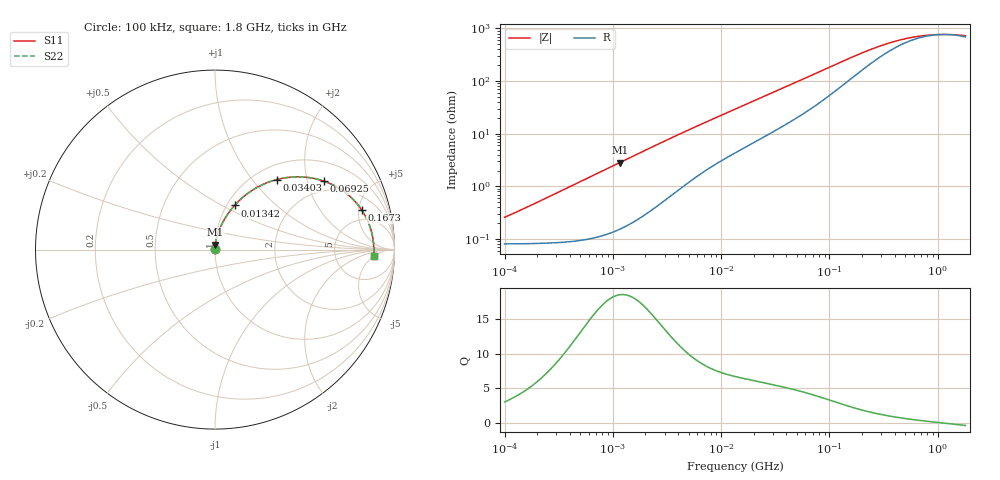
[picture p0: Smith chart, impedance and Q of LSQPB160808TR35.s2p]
! LSQPB160808TR35  S-PARAMETER MODEL  ( General Type )
! Model Generated by TAIYO YUDEN Corporation (http://www.ty-top.com)
! Version 4.0
! TAIYO YUDEN Control No. 100810NF18SB-HKC
! Copyright(c) 2007 TAIYO YUDEN CO.,LTD. All Rights Reserved.
! Product Description (link to TY-COMPAS)
! https://ds.yuden.co.jp/TYCOMPAS/or/detail?pn=LSQPB160808TR35M&u=M
! Products Name : Inductors
! Characteristics :
!  Inductance : 0.35 uH , SRF(min) : 300 MHz , DC Resistance(max) : 0.104 Ohm
!  Rated Current : Saturation :1400 mA , Temp Rise : 810 mA (40 degC)
!  Case Size : 1.6 x 0.8 / 0.063 x 0.031 [mm/inch] , Thickness : 0.8 / 0.031 [mm/inch]
!  (Conditions: Temperature = 25 degC , DC Bias Current/Voltage = 0A / 0V)
! External Node Assignments :
!  1  o---GGG---o  2
! GND o---------o GND
! Frequency Range : 0.1MHz  -  1800MHz  [ 402 STEP ]
# MHz S RI R 50
! Freq[MHz].  S11 Real  S11 Imag  S21 Real  S21 Imag  S12 Real  S12 Imag  S22 Real  S22 Imag
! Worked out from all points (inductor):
!   401 points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, 100 kHz to 1.8 GHz, reference 50 ohm
!   read as one part in series: L = 390 nH near 105 kHz
!   highest Q = 18.5 at 1.158 MHz (marker M1), where L = 389 nH
!   self-resonance near 1.142 GHz
!   S11 on the Smith chart (normalised r, x): 100 kHz: 1.00, +0.00; 13.42 MHz: 1.09, +0.58; 34.03 MHz: 1.25, +1.34; 69.25 MHz: 1.62, +2.54; 167.3 MHz: 3.43, +5.36; 1.8 GHz: 15, -5
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0.1  0.000811 0.00245  0.9992 -0.00245  0.9992 -0.00245  0.000811 0.00245
0.163216  0.00083 0.00399  0.9992 -0.00399  0.9992 -0.00399  0.00083 0.00399
0.516129  0.00111 0.0126  0.9989 -0.0126  0.9989 -0.0126  0.00111 0.0126
1.158292  0.00233 0.0282  0.9977 -0.0282  0.9977 -0.0282  0.00233 0.0282
2.66389  0.00851 0.0635  0.9915 -0.0635  0.9915 -0.0635  0.00851 0.0635
4.347904  0.0197 0.1  0.9803 -0.1  0.9803 -0.1  0.0197 0.1
6.757206  0.0403 0.1463  0.9597 -0.1463  0.9597 -0.1463  0.0403 0.1463
9.75753  0.0699 0.1957  0.9301 -0.1957  0.9301 -0.1957  0.0699 0.1957
13.41641  0.1094 0.2463  0.8906 -0.2463  0.8906 -0.2463  0.1094 0.2463
21.36789  0.2015 0.3265  0.7985 -0.3265  0.7985 -0.3265  0.2015 0.3265
34.03197  0.3427 0.39  0.6573 -0.39  0.6573 -0.39  0.3427 0.39
49.1428  0.4793 0.4052  0.5207 -0.4052  0.5207 -0.4052  0.4793 0.4052
69.24595  0.6064 0.3816  0.3936 -0.3816  0.3936 -0.3816  0.6064 0.3816
86.32529  0.678 0.3495  0.322 -0.3495  0.322 -0.3495  0.678 0.3495
107.6172  0.7372 0.309  0.2628 -0.309  0.2628 -0.309  0.7372 0.309
167.2511  0.8167 0.2218  0.1833 -0.2218  0.1833 -0.2218  0.8167 0.2218
235.6695  0.8502 0.1616  0.1498 -0.1616  0.1498 -0.1616  0.8502 0.1616
357.3983  0.871 0.1033  0.129 -0.1033  0.129 -0.1033  0.871 0.1033
542.0029  0.8803 0.0593  0.1197 -0.0593  0.1197 -0.0593  0.8803 0.0593
802.0705  0.8839 0.0263  0.1161 -0.0263  0.1161 -0.0263  0.8839 0.0263
1186.925  0.8849 -0.0028  0.1151 0.0028  0.1151 0.0028  0.8849 -0.0028
1800  0.8837 -0.0343  0.1163 0.0343  0.1163 0.0343  0.8837 -0.0343
